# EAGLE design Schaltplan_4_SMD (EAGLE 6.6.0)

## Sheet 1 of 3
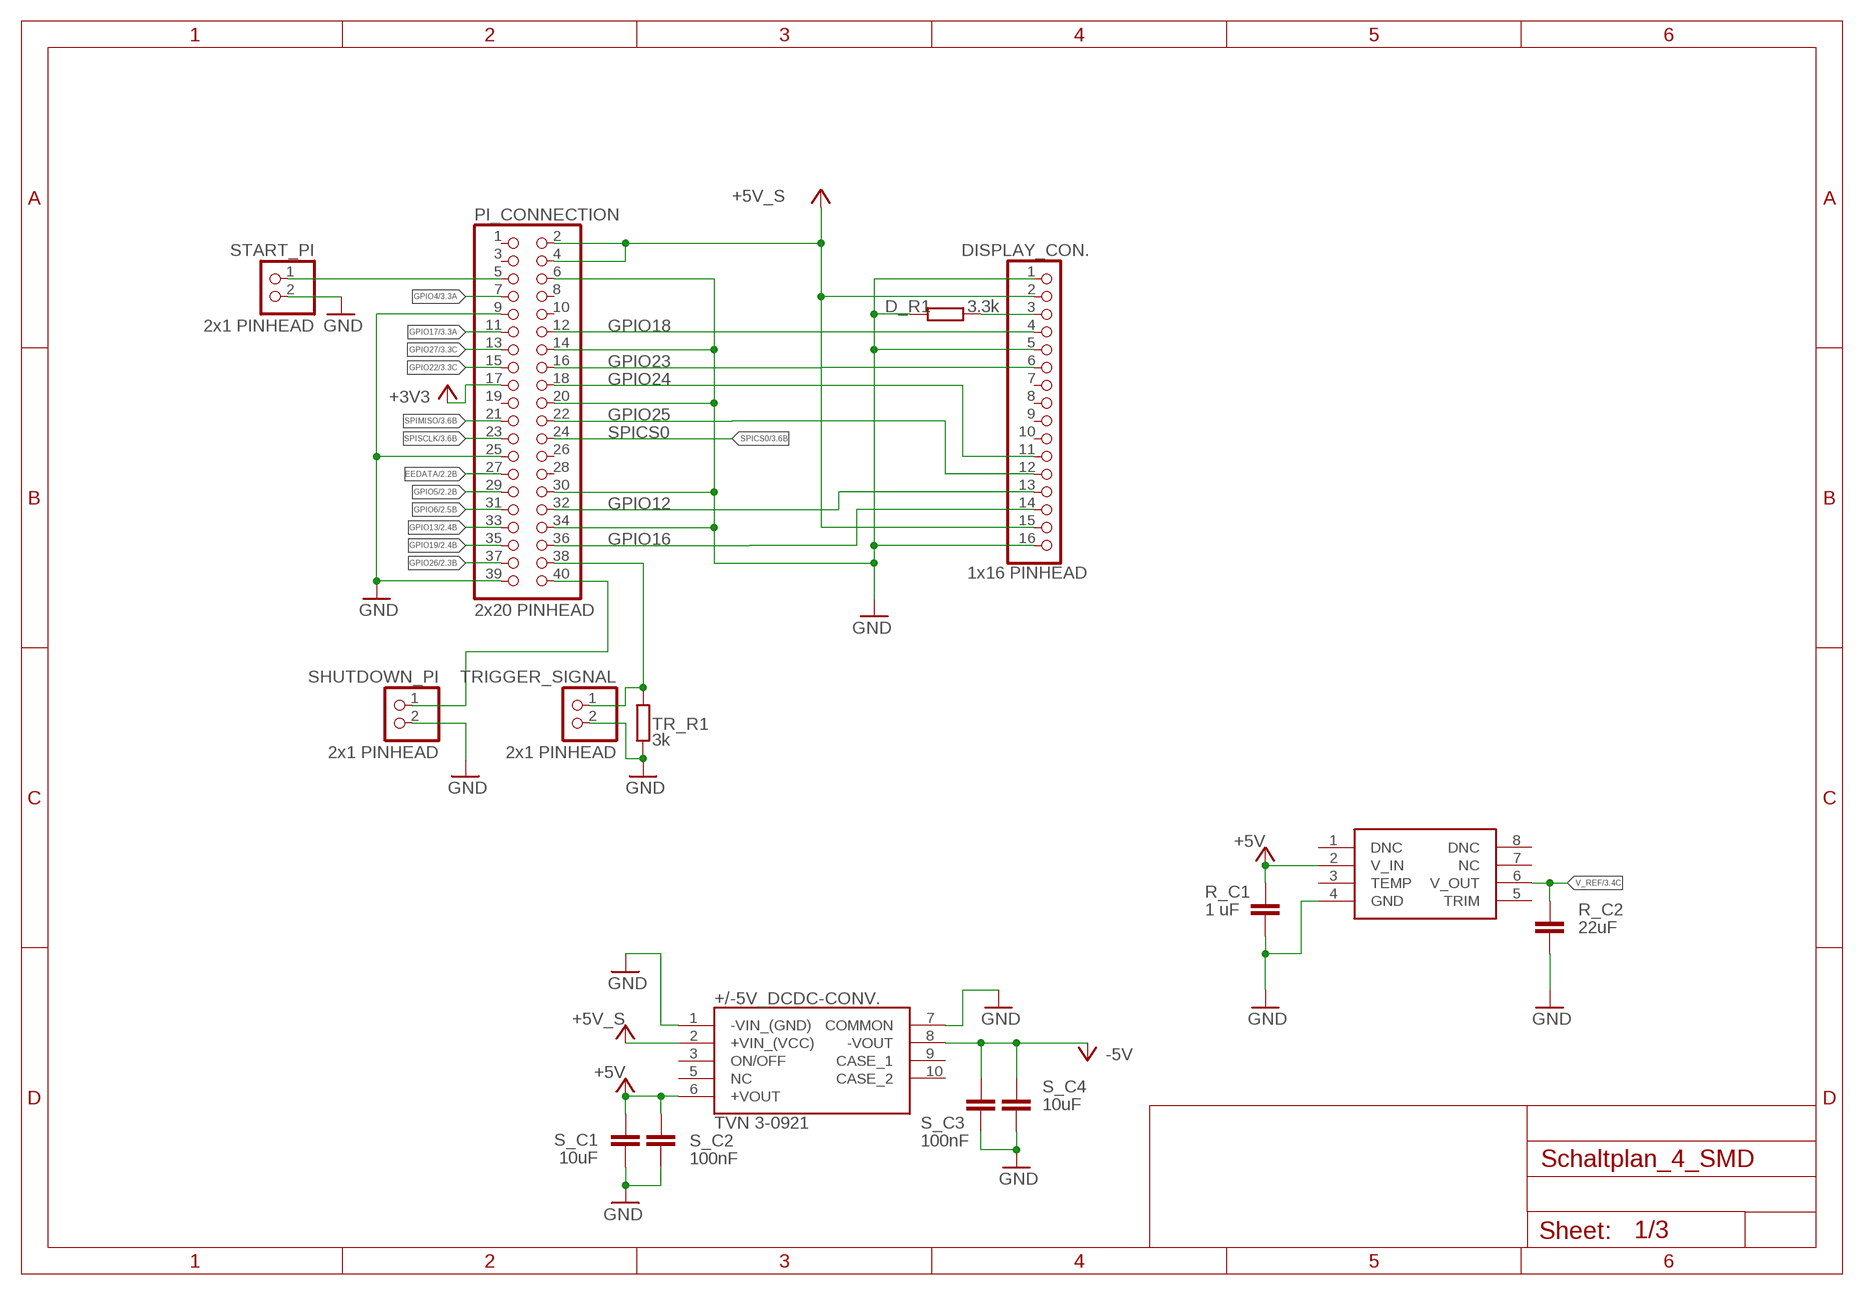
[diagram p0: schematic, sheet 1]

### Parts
+/-5V_DCDC-CONV.  TVN 3-0921  TVN_3-1223  [TVN32419]
D_R1  3.3k  R-EU_0207/10  [0207/10]
DISPLAY_CON.  1x16 PINHEAD  PINHD-1X16  [1X16]
PI_CONNECTION  2x20 PINHEAD  PINHD-2X20  [2X20]
R_C1  1 uF  C-EU025-030X050  [C025-030X050]
R_C2  22uF  C-EU025-030X050  [C025-030X050]
REF_VOLTAGE  REF5020  [SOIC8]
S_C1  10uF  C-EU025-030X050  [C025-030X050]
S_C2  100nF  C-EU025-030X050  [C025-030X050]
S_C3  100nF  C-EU025-030X050  [C025-030X050]
S_C4  10uF  C-EU025-030X050  [C025-030X050]
SHUTDOWN_PI  2x1 PINHEAD  PINHD-1X2  [1X02]
START_PI  2x1 PINHEAD  PINHD-1X2  [1X02]
TR_R1  3k  R-EU_0207/10  [0207/10]
TRIGGER_SIGNAL  2x1 PINHEAD  PINHD-1X2  [1X02]

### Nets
+3V3: PI_CONNECTION.17 ; also sheet 3
+5V: +/-5V_DCDC-CONV..6(+VOUT) R_C1.1 REF_VOLTAGE.2(V_IN) S_C1.1 S_C2.1 ; also sheet 2,3
+5V_SUPPLY: +/-5V_DCDC-CONV..2(+VIN_(VCC)) DISPLAY_CON..2 DISPLAY_CON..15 PI_CONNECTION.2 PI_CONNECTION.4 ; supply symbol labelled +5V_S
-5V: +/-5V_DCDC-CONV..8(-VOUT) S_C3.1 S_C4.2 ; also sheet 2,3
EEDATA: PI_CONNECTION.27 ; also sheet 2
GND: +/-5V_DCDC-CONV..1(-VIN_(GND)) +/-5V_DCDC-CONV..7(COMMON) D_R1.1 DISPLAY_CON..1 DISPLAY_CON..5 DISPLAY_CON..16 PI_CONNECTION.6 PI_CONNECTION.9 PI_CONNECTION.14 PI_CONNECTION.20 PI_CONNECTION.25 PI_CONNECTION.30 PI_CONNECTION.34 PI_CONNECTION.39 R_C1.2 R_C2.2 REF_VOLTAGE.4(GND) S_C1.2 S_C2.2 S_C3.2 S_C4.1 SHUTDOWN_PI.2 START_PI.2 TR_R1.1 TRIGGER_SIGNAL.2 ; also sheet 2,3
GPIO4: PI_CONNECTION.7 ; also sheet 3
GPIO5: PI_CONNECTION.29 ; also sheet 2
GPIO6: PI_CONNECTION.31 ; also sheet 2
GPIO12: DISPLAY_CON..13 PI_CONNECTION.32
GPIO13: PI_CONNECTION.33 ; also sheet 2
GPIO16: DISPLAY_CON..14 PI_CONNECTION.36
GPIO17: PI_CONNECTION.11 ; also sheet 3
GPIO18: DISPLAY_CON..4 PI_CONNECTION.12
GPIO19: PI_CONNECTION.35 ; also sheet 2
GPIO20: PI_CONNECTION.38 TR_R1.2 TRIGGER_SIGNAL.1
GPIO21: PI_CONNECTION.40 SHUTDOWN_PI.1
GPIO22: PI_CONNECTION.15 ; also sheet 3
GPIO23: DISPLAY_CON..6 PI_CONNECTION.16
GPIO24: DISPLAY_CON..11 PI_CONNECTION.18
GPIO25: DISPLAY_CON..12 PI_CONNECTION.22
GPIO26: PI_CONNECTION.37 ; also sheet 2
GPIO27: PI_CONNECTION.13 ; also sheet 3
N$3: D_R1.2 DISPLAY_CON..3
SCL1: PI_CONNECTION.5 START_PI.1
SPICS0: PI_CONNECTION.24 ; also sheet 3
SPIMISO: PI_CONNECTION.21 ; also sheet 3
SPISCLK: PI_CONNECTION.23 ; also sheet 3
V_REF: R_C2.1 REF_VOLTAGE.6(V_OUT) ; also sheet 3
Unconnected: +/-5V_DCDC-CONV..3(ON/OFF) +/-5V_DCDC-CONV..5(NC) +/-5V_DCDC-CONV..9(CASE_1) +/-5V_DCDC-CONV..10(CASE_2) DISPLAY_CON..7 DISPLAY_CON..8 DISPLAY_CON..9 DISPLAY_CON..10 PI_CONNECTION.1 PI_CONNECTION.3 PI_CONNECTION.8 PI_CONNECTION.10 PI_CONNECTION.19 PI_CONNECTION.26 PI_CONNECTION.28 REF_VOLTAGE.1(DNC) REF_VOLTAGE.3(TEMP) REF_VOLTAGE.5(TRIM) REF_VOLTAGE.7(NC) REF_VOLTAGE.8(DNC)

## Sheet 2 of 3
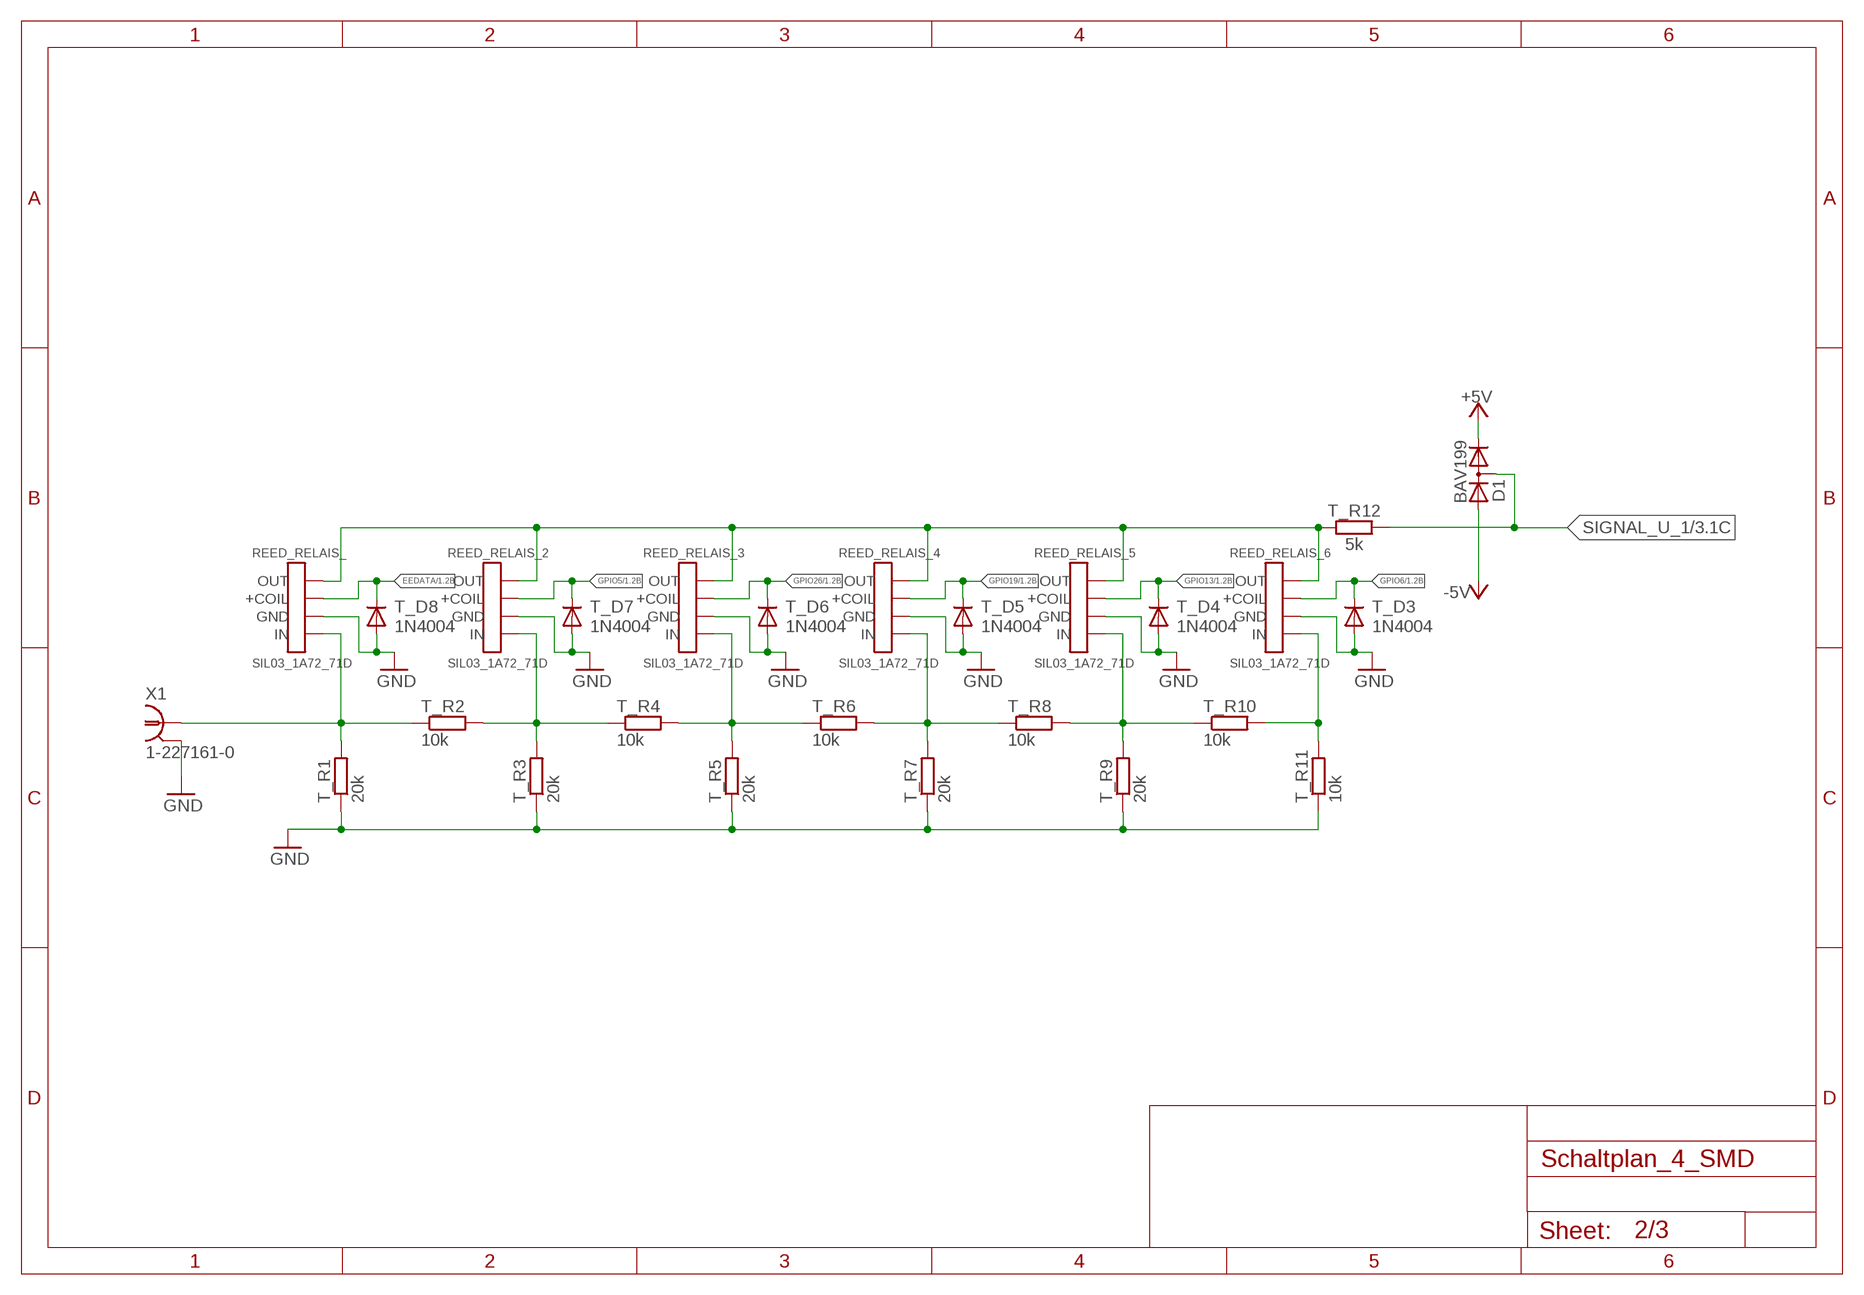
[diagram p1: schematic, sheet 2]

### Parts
D1  BAV199  [SOT23]
REED_RELAIS_  SIL03_1A72_71D  REED_REALIS_SIL03_1A72_71D  [REED_RELAIS_SIL03_1A72_71D]
REED_RELAIS_2  SIL03_1A72_71D  REED_REALIS_SIL03_1A72_71D  [REED_RELAIS_SIL03_1A72_71D]
REED_RELAIS_3  SIL03_1A72_71D  REED_REALIS_SIL03_1A72_71D  [REED_RELAIS_SIL03_1A72_71D]
REED_RELAIS_4  SIL03_1A72_71D  REED_REALIS_SIL03_1A72_71D  [REED_RELAIS_SIL03_1A72_71D]
REED_RELAIS_5  SIL03_1A72_71D  REED_REALIS_SIL03_1A72_71D  [REED_RELAIS_SIL03_1A72_71D]
REED_RELAIS_6  SIL03_1A72_71D  REED_REALIS_SIL03_1A72_71D  [REED_RELAIS_SIL03_1A72_71D]
T_D3  1N4004  BAV17  [DO35-10]
T_D4  1N4004  BAV17  [DO35-10]
T_D5  1N4004  BAV17  [DO35-10]
T_D6  1N4004  BAV17  [DO35-10]
T_D7  1N4004  BAV17  [DO35-10]
T_D8  1N4004  BAV17  [DO35-10]
T_R1  20k  R-EU_0207/10  [0207/10]
T_R2  10k  R-EU_0207/10  [0207/10]
T_R3  20k  R-EU_0207/10  [0207/10]
T_R4  10k  R-EU_0207/10  [0207/10]
T_R5  20k  R-EU_0207/10  [0207/10]
T_R6  10k  R-EU_0207/10  [0207/10]
T_R7  20k  R-EU_0207/10  [0207/10]
T_R8  10k  R-EU_0207/10  [0207/10]
T_R9  20k  R-EU_0207/10  [0207/10]
T_R10  10k  R-EU_0207/10  [0207/10]
T_R11  10k  R-EU_0207/10  [0207/10]
T_R12  5k  R-EU_0207/10  [0207/10]
X1  1-227161-0  [AMP_227161]

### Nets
+5V: D1.2(C) ; also sheet 1,3
-5V: D1.1(A) ; also sheet 1,3
EEDATA: REED_RELAIS_.P$2(+COIL) T_D8.C ; also sheet 1
GND: REED_RELAIS_2.P$3(GND) REED_RELAIS_3.P$3(GND) REED_RELAIS_4.P$3(GND) REED_RELAIS_5.P$3(GND) REED_RELAIS_6.P$3(GND) REED_RELAIS_.P$3(GND) T_D3.A T_D4.A T_D5.A T_D6.A T_D7.A T_D8.A T_R1.1 T_R3.1 T_R5.1 T_R7.1 T_R9.1 T_R11.1 X1.2 ; also sheet 1,3
GPIO5: REED_RELAIS_2.P$2(+COIL) T_D7.C ; also sheet 1
GPIO6: REED_RELAIS_6.P$2(+COIL) T_D3.C ; also sheet 1
GPIO13: REED_RELAIS_5.P$2(+COIL) T_D4.C ; also sheet 1
GPIO19: REED_RELAIS_4.P$2(+COIL) T_D5.C ; also sheet 1
GPIO26: REED_RELAIS_3.P$2(+COIL) T_D6.C ; also sheet 1
N$2: REED_RELAIS_2.P$1(OUT) REED_RELAIS_3.P$1(OUT) REED_RELAIS_4.P$1(OUT) REED_RELAIS_5.P$1(OUT) REED_RELAIS_6.P$1(OUT) REED_RELAIS_.P$1(OUT) T_R12.1
N$42: REED_RELAIS_2.P$4(IN) T_R2.2 T_R3.2 T_R4.1
N$43: REED_RELAIS_3.P$4(IN) T_R4.2 T_R5.2 T_R6.1
N$44: REED_RELAIS_4.P$4(IN) T_R6.2 T_R7.2 T_R8.1
N$45: REED_RELAIS_5.P$4(IN) T_R8.2 T_R9.2 T_R10.1
N$46: REED_RELAIS_6.P$4(IN) T_R10.2 T_R11.2
SIGNAL_U_0: REED_RELAIS_.P$4(IN) T_R1.2 T_R2.1 X1.1
SIGNAL_U_1: D1.3(AC) T_R12.2 ; also sheet 3

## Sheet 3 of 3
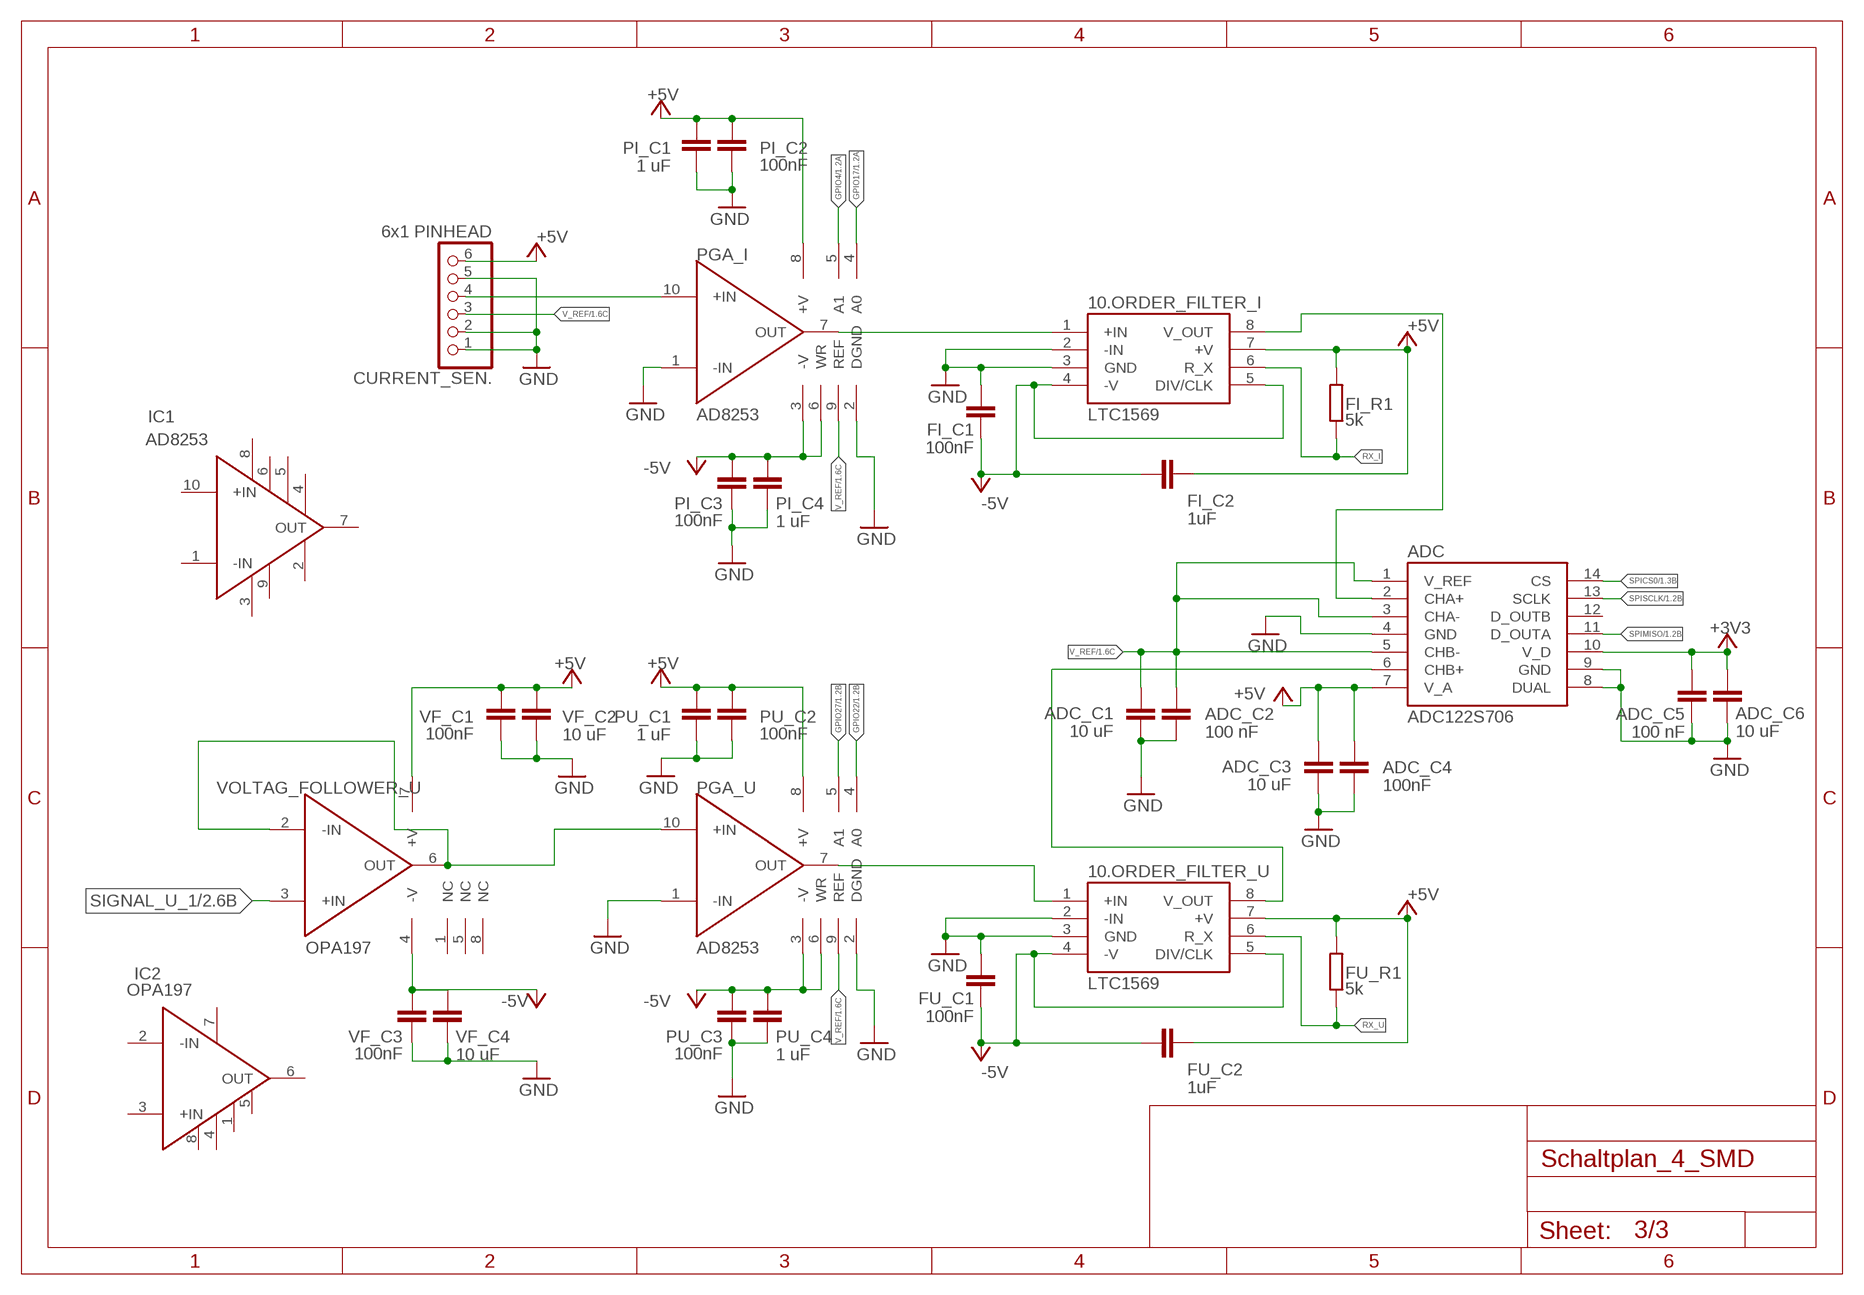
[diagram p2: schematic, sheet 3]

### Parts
10.ORDER_FILTER_I  LTC1569  [SO-08]
10.ORDER_FILTER_U  LTC1569  [SO-08]
ADC  ADC122S706  [TSSOP14]
ADC_C1  10 uF  C-EU025-030X050  [C025-030X050]
ADC_C2  100 nF  C-EU025-030X050  [C025-030X050]
ADC_C3  10 uF  C-EU025-030X050  [C025-030X050]
ADC_C4  100nF  C-EU025-030X050  [C025-030X050]
ADC_C5  100 nF  C-EU025-030X050  [C025-030X050]
ADC_C6  10 uF  C-EU025-030X050  [C025-030X050]
CURRENT_SEN.  6x1 PINHEAD  PINHD-1X6  [1X06]
FI_C1  100nF  C-EU025-030X050  [C025-030X050]
FI_C2  1uF  C-EU025-030X050  [C025-030X050]
FI_R1  5k  R-EU_0207/10  [0207/10]
FU_C1  100nF  C-EU025-030X050  [C025-030X050]
FU_C2  1uF  C-EU025-030X050  [C025-030X050]
FU_R1  5k  R-EU_0207/10  [0207/10]
IC1  AD8253  [MSOP10]
IC2  OPA197  [UMAX8]
PGA_I  AD8253  [MSOP10]
PGA_U  AD8253  [MSOP10]
PI_C1  1 uF  C-EU025-030X050  [C025-030X050]
PI_C2  100nF  C-EU025-030X050  [C025-030X050]
PI_C3  100nF  C-EU025-030X050  [C025-030X050]
PI_C4  1 uF  C-EU025-030X050  [C025-030X050]
PU_C1  1 uF  C-EU025-030X050  [C025-030X050]
PU_C2  100nF  C-EU025-030X050  [C025-030X050]
PU_C3  100nF  C-EU025-030X050  [C025-030X050]
PU_C4  1 uF  C-EU025-030X050  [C025-030X050]
VF_C1  100nF  C-EU025-030X050  [C025-030X050]
VF_C2  10 uF  C-EU025-030X050  [C025-030X050]
VF_C3  100nF  C-EU025-030X050  [C025-030X050]
VF_C4  10 uF  C-EU025-030X050  [C025-030X050]
VOLTAG_FOLLOWER_U  OPA197  [UMAX8]

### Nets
+3V3: ADC.10(V_D) ADC_C5.1 ADC_C6.1 ; also sheet 1
+5V: 10.ORDER_FILTER_I.7(+V) 10.ORDER_FILTER_U.7(+V) ADC.7(V_A) ADC_C3.1 ADC_C4.1 CURRENT_SEN..6 FI_C2.2 FI_R1.2 FU_C2.2 FU_R1.2 PGA_I.8(+V) PGA_U.8(+V) PI_C1.2 PI_C2.1 PU_C1.2 PU_C2.1 VF_C1.1 VF_C2.2 VOLTAG_FOLLOWER_U.7(+V) ; also sheet 1,2
-5V: 10.ORDER_FILTER_I.4(-V) 10.ORDER_FILTER_I.5(DIV/CLK) 10.ORDER_FILTER_U.4(-V) 10.ORDER_FILTER_U.5(DIV/CLK) FI_C1.1 FI_C2.1 FU_C1.1 FU_C2.1 PGA_I.3(-V) PGA_I.6(WR) PGA_U.3(-V) PGA_U.6(WR) PI_C3.1 PI_C4.2 PU_C3.1 PU_C4.2 VF_C3.1 VF_C4.2 VOLTAG_FOLLOWER_U.4(-V) ; also sheet 1,2
GND: 10.ORDER_FILTER_I.2(-IN) 10.ORDER_FILTER_I.3(GND) 10.ORDER_FILTER_U.2(-IN) 10.ORDER_FILTER_U.3(GND) ADC.4(GND) ADC.8(DUAL) ADC.9(GND) ADC_C1.2 ADC_C2.2 ADC_C3.2 ADC_C4.2 ADC_C5.2 ADC_C6.2 CURRENT_SEN..1 CURRENT_SEN..2 CURRENT_SEN..5 FI_C1.2 FU_C1.2 PGA_I.1(-IN) PGA_I.2(DGND) PGA_U.1(-IN) PGA_U.2(DGND) PI_C1.1 PI_C2.2 PI_C3.2 PI_C4.1 PU_C1.1 PU_C2.2 PU_C3.2 PU_C4.1 VF_C1.2 VF_C2.1 VF_C3.2 VF_C4.1 ; also sheet 1,2
GPIO4: PGA_I.5(A1) ; also sheet 1
GPIO17: PGA_I.4(A0) ; also sheet 1
GPIO22: PGA_U.4(A0) ; also sheet 1
GPIO27: PGA_U.5(A1) ; also sheet 1
RX_I: 10.ORDER_FILTER_I.6(R_X) FI_R1.1
RX_U: 10.ORDER_FILTER_U.6(R_X) FU_R1.1
SIGNAL_I_0: CURRENT_SEN..4 PGA_I.10(+IN)
SIGNAL_I_1: 10.ORDER_FILTER_I.1(+IN) PGA_I.7(OUT)
SIGNAL_I_2: 10.ORDER_FILTER_I.8(V_OUT) ADC.2(CHA+)
SIGNAL_U_1: VOLTAG_FOLLOWER_U.3(+IN) ; also sheet 2
SIGNAL_U_2: PGA_U.10(+IN) VOLTAG_FOLLOWER_U.2(-IN) VOLTAG_FOLLOWER_U.6(OUT)
SIGNAL_U_3: 10.ORDER_FILTER_U.1(+IN) PGA_U.7(OUT)
SIGNAL_U_4: 10.ORDER_FILTER_U.8(V_OUT) ADC.6(CHB+)
SPICS0: ADC.14(CS) ; also sheet 1
SPIMISO: ADC.11(D_OUTA) ; also sheet 1
SPISCLK: ADC.13(SCLK) ; also sheet 1
V_REF: ADC.1(V_REF) ADC.3(CHA-) ADC.5(CHB-) ADC_C1.1 ADC_C2.1 CURRENT_SEN..3 PGA_I.9(REF) PGA_U.9(REF) ; also sheet 1
Unconnected: ADC.12(D_OUTB) IC1.1(-IN) IC1.4(A0) IC1.5(A1) IC1.6(WR) IC1.7(OUT) IC1.9(REF) IC1.10(+IN) IC2.1(NC) IC2.2(-IN) IC2.3(+IN) IC2.5(NC) IC2.6(OUT) IC2.8(NC) VOLTAG_FOLLOWER_U.1(NC) VOLTAG_FOLLOWER_U.5(NC) VOLTAG_FOLLOWER_U.8(NC)

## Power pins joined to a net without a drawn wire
+V: IC1.8(+V) IC2.7(+V)
-V: IC1.3(-V) IC2.4(-V)
DGND: IC1.2(DGND)

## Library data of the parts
10.ORDER_FILTER_I 10.ORDER_FILTER_U = ref-packages:LTC1569
+/-5V_DCDC-CONV. = TVN_3-1223:TVN_3-1223: Isolated DC/DC Converters 3W 9-18Vin SIP-8 +/-15Vout +/-100mA Source: Datasheet; ALLIED_NUMBER: 71099550; ALLIED_PRICE-STOCK: https://www.alliedelec.com/traco-power-tvn-3-1223/71099550/; DESCRIPTION: Isolated DC/DC Converters 3W 9-18Vin SIP-8 +/-15Vout +/-100mA; HEIGHT: 11mm; MANUFACTURER_NAME: Traco Power; MANUFACTURER_PART_NUMBER: TVN 3-1223; MOUSER_PART_NUMBER: 495-TVN3-1223; MOUSER_PRICE-STOCK: https://www.mouser.com/Search/Refine.aspx?Keyword=495-TVN3-1223; RS_PART_NUMBER: 1466094; RS_PRICE-STOCK: https://uk.rs-online.com/web/p/products/1466094
ADC = ref-packages:ADC122S706
ADC_C1-ADC_C6 FI_C1 FI_C2 FU_C1 FU_C2 PI_C1-PI_C4 PU_C1-PU_C4 R_C1 R_C2 S_C1-S_C4 VF_C1-VF_C4 = rcl:C-EU: CAPACITOR, European symbol
CURRENT_SEN. = pinhead:PINHD-1X6: PIN HEADER
D1 = diode:BAV199: DIODE low-leakage double diode
D_R1 FI_R1 FU_R1 T_R1-T_R12 TR_R1 = rcl:R-EU_: RESISTOR, European symbol
DISPLAY_CON. = pinhead:PINHD-1X16: PIN HEADER
IC1 = Schaltplan_4_SMD:AD8253
IC2 = Schaltplan_4_SMD:OPA197
PGA_I PGA_U = ref-packages:AD8253
PI_CONNECTION = pinhead:PINHD-2X20: PIN HEADER
REED_RELAIS_ REED_RELAIS_2-REED_RELAIS_6 = OWN_Library:REED_REALIS_SIL03_1A72_71D
REF_VOLTAGE = ref-packages:REF5020
SHUTDOWN_PI START_PI TRIGGER_SIGNAL = pinhead:PINHD-1X2: PIN HEADER
T_D3-T_D8 = diode:BAV17: DIODE
VOLTAG_FOLLOWER_U = ref-packages:OPA197
X1 = con-coax:?227161*: JACK, RIGHT ANGLE, 50 OHM, PCB, BNC; MF: TYCO ELECTRONICS; MPN: 1-227161; OC_FARNELL: unknown; OC_NEWARK: 33B3200

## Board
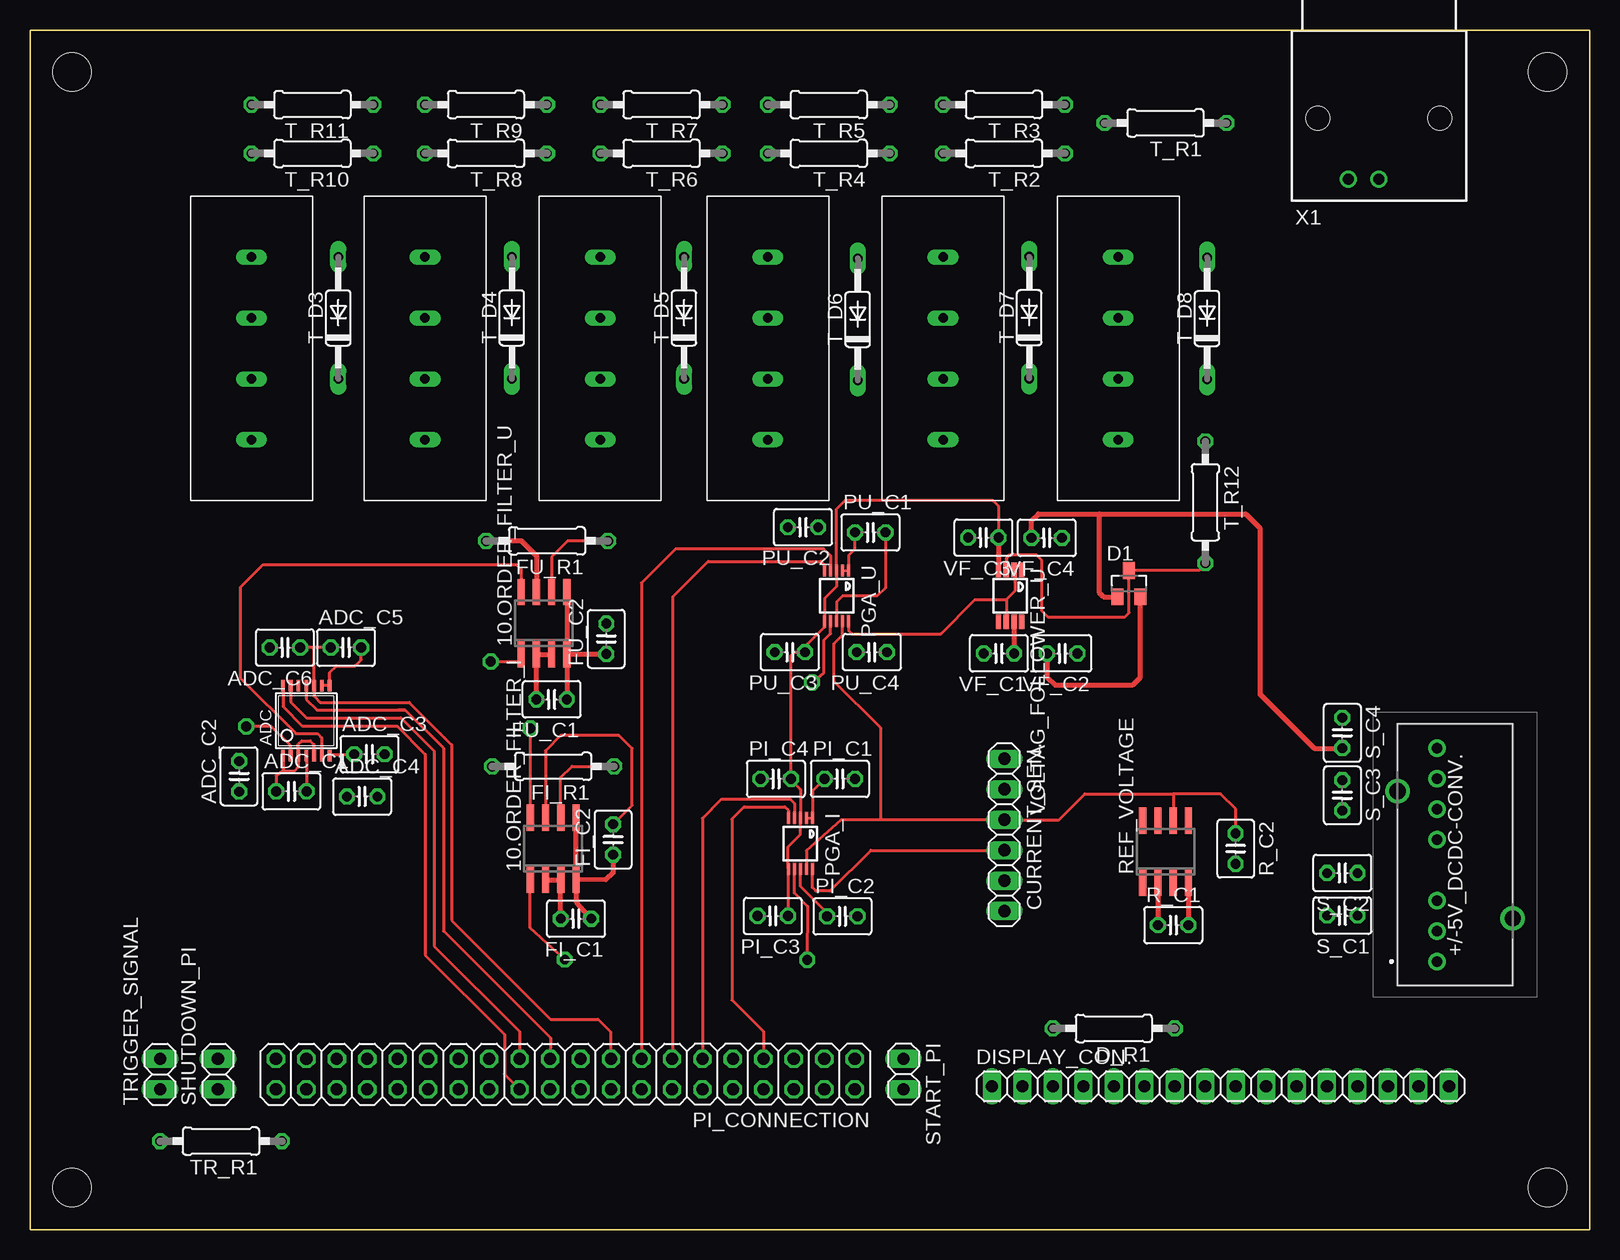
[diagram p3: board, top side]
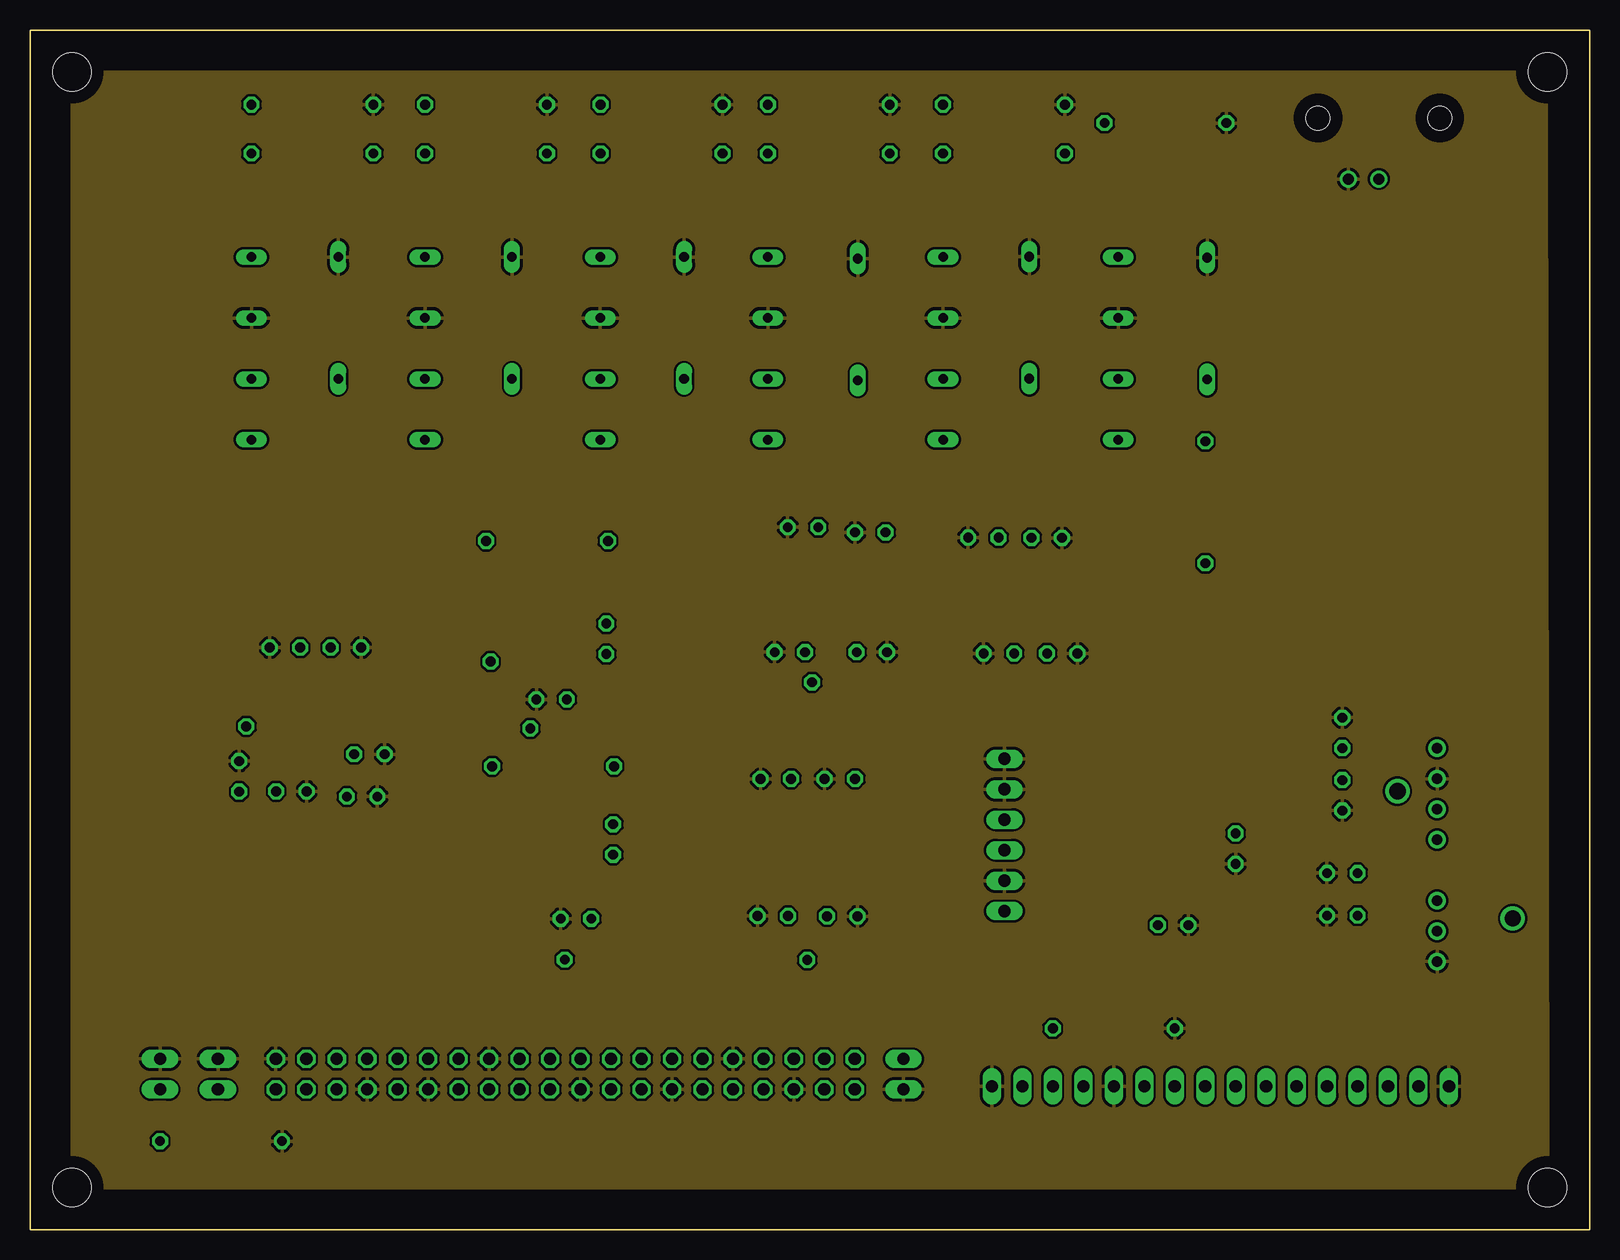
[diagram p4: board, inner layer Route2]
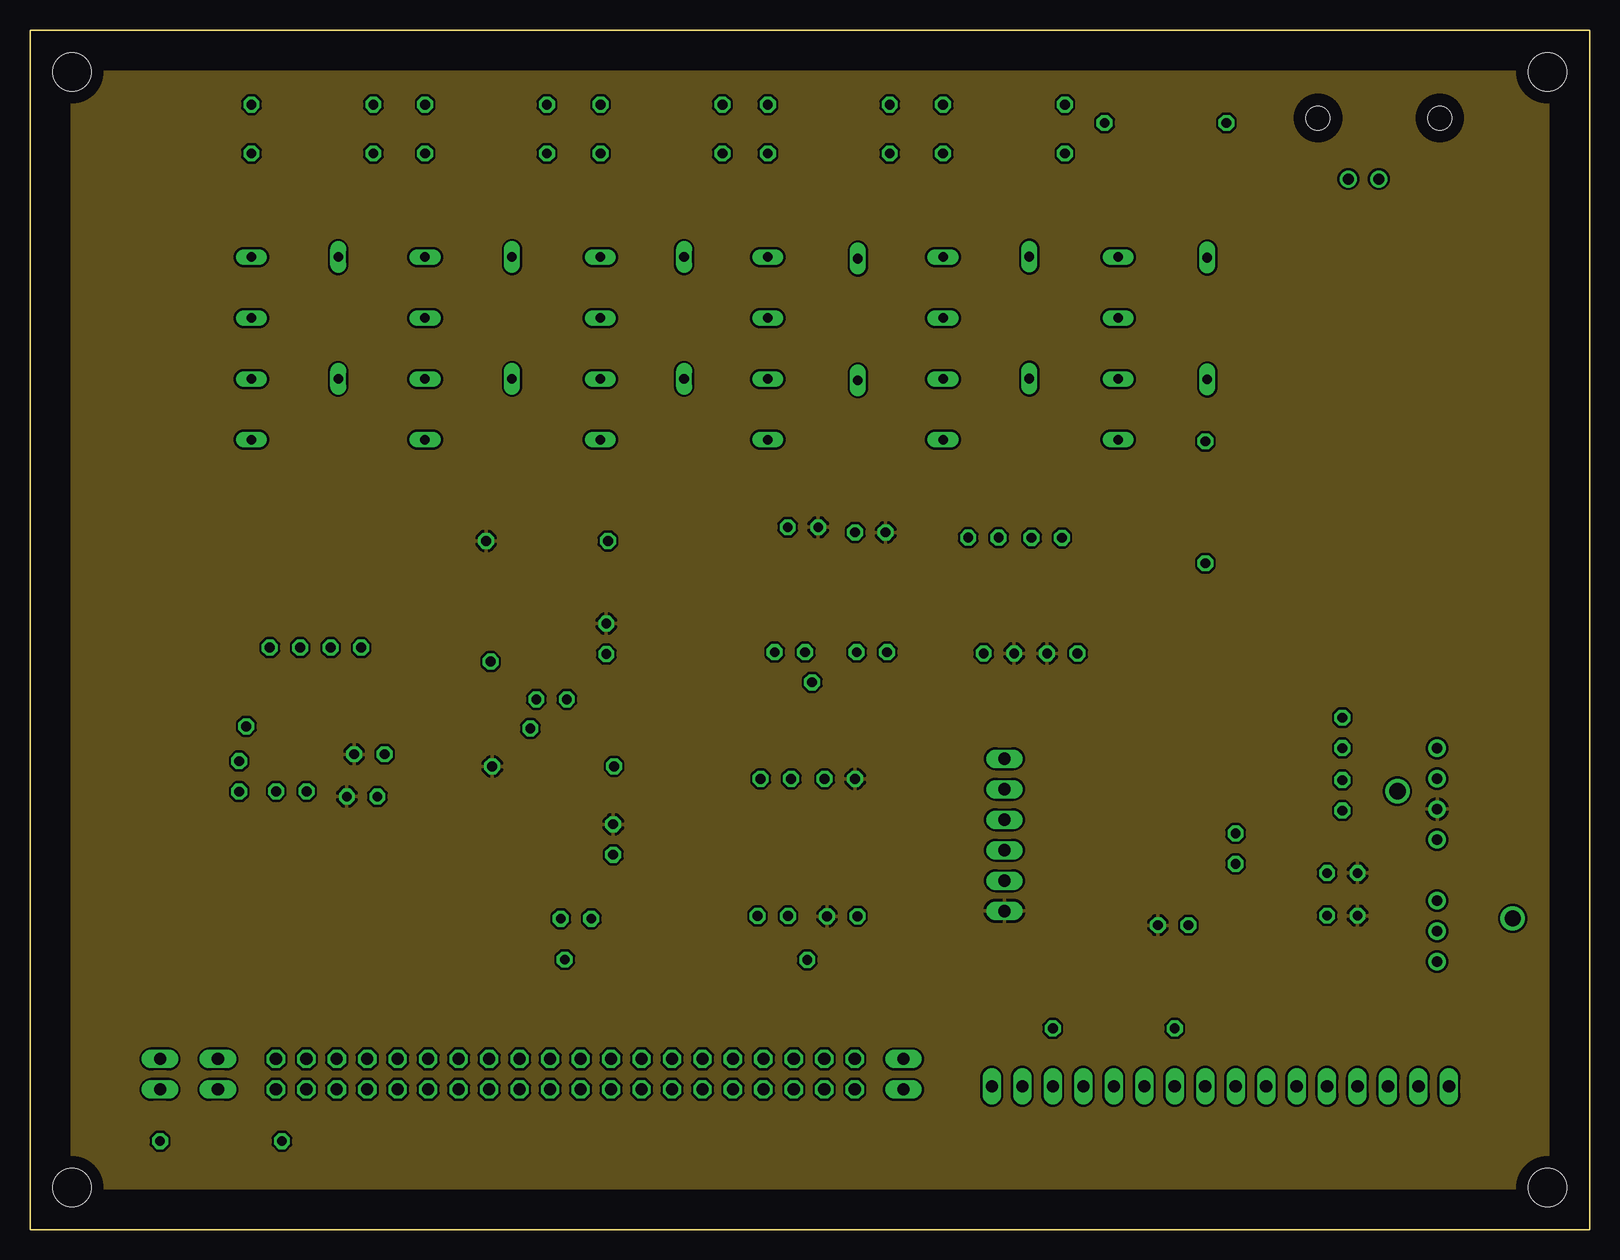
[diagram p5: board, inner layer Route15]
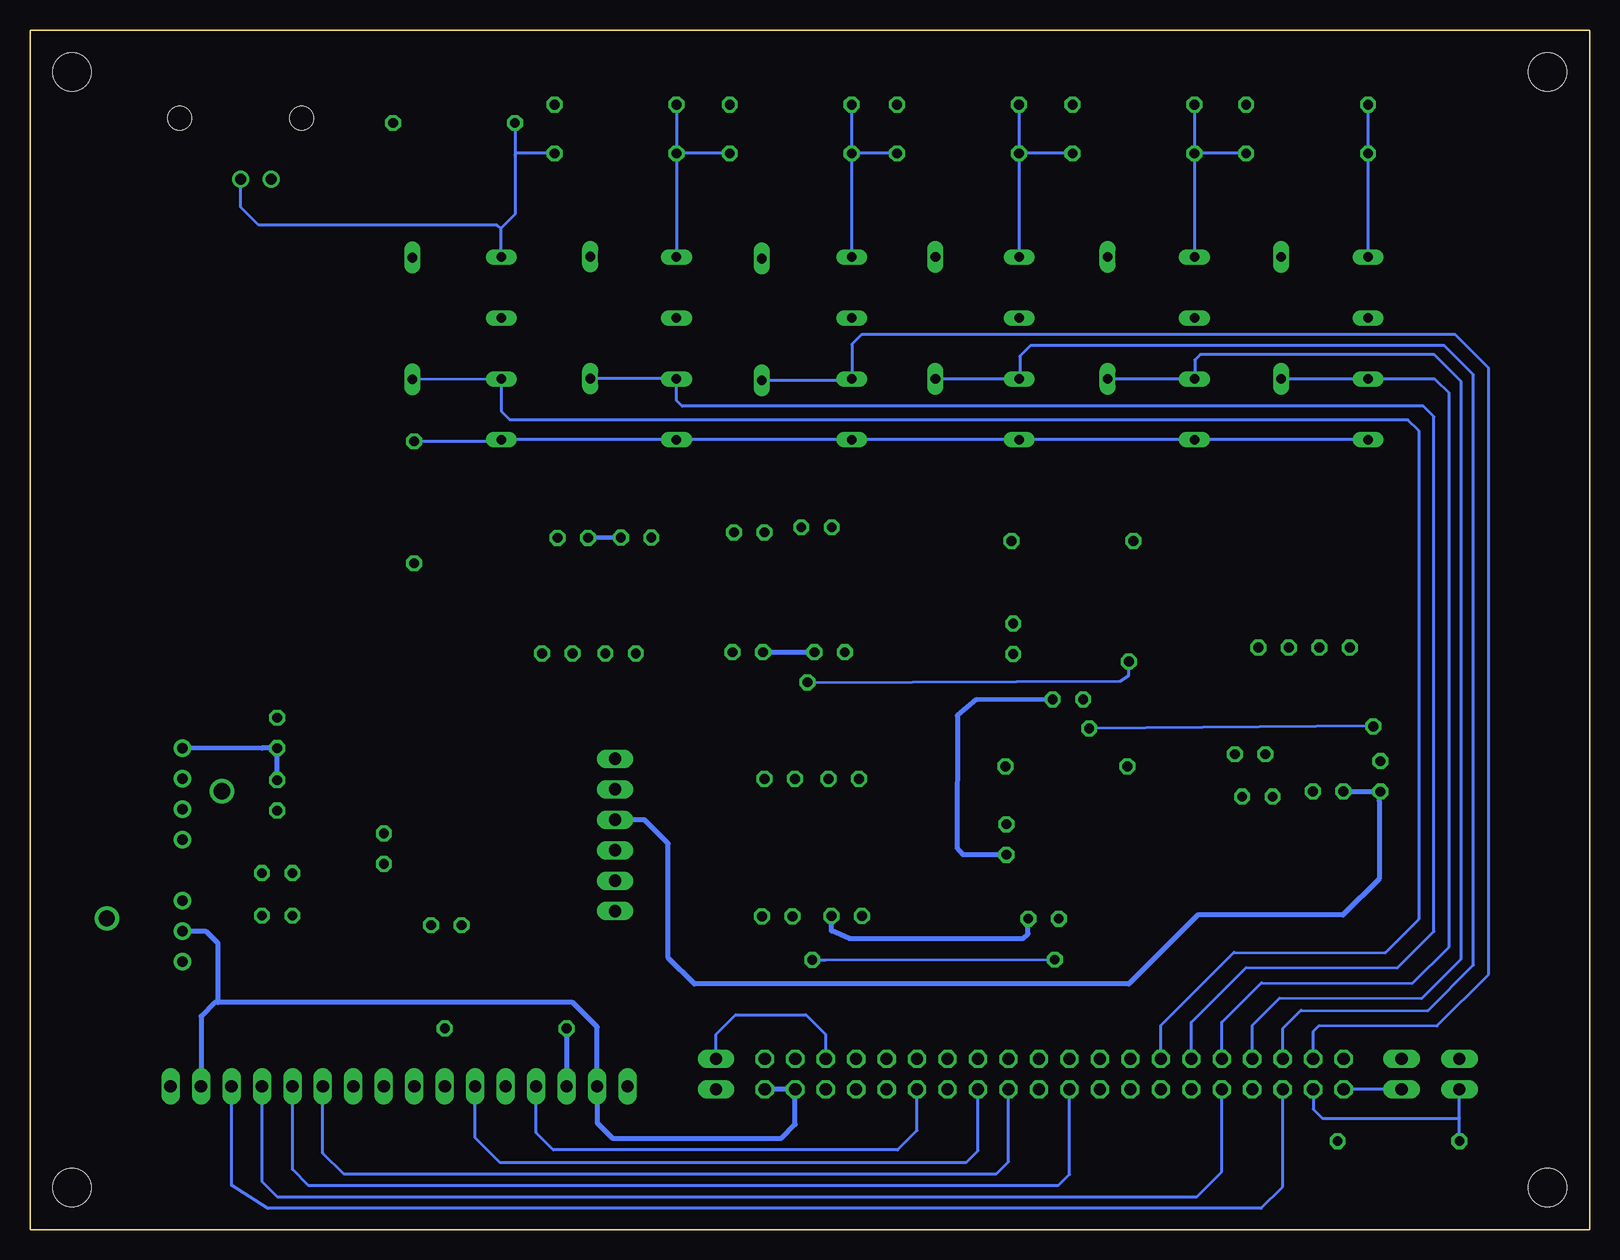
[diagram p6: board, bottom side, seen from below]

Size 130 x 100 mm. Coordinates in mm from the lower left corner, seen from the top.
Outline: 0,0 0,100 130,100 130,0 0,0
Copper layers ((1*2)+(15*16)): Top 0.035mm / dielectric 0.3mm / Route2 0.035mm / dielectric 0.3mm / Route15 0.035mm / dielectric 0.3mm / Bottom 0.035mm
Design rules "default *": minimum track width 10mil, minimum drill 24mil, track to track 8mil, track to pad 2mil, pad to pad 2mil, via to via 8mil, smd to smd 2mil, copper to edge 40mil, drill to drill 8mil, minimum pad ring 10mil, minimum via ring 8mil, stop-mask expansion 4mil, vias tented up to drill 0mil, thermal gap 10mil
Holes 3.2 mm at 3.5,3.5 126.5,96.5 126.5,3.5 3.5,96.5

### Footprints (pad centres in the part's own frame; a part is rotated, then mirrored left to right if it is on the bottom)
SO-08 = smd 0.6 x 2.2: 1 -1.905,-2.6; 2 -0.635,-2.6; 3 0.635,-2.6; 4 1.905,-2.6; 5 1.905,2.6; 6 0.635,2.6; 7 -0.635,2.6; 8 -1.905,2.6
TVN32419 = drill 0.89 pad 1.446: 1 -8.9,1.5; 2 -6.36,1.5; 3 -3.82,1.5; 5 1.26,1.5; 6 3.8,1.5; 7 6.34,1.5; 8 8.88,1.5 | drill 1.35 pad 2.025: 9 -5.3,-4.8; 10 5.3,4.8
TSSOP14 = smd 0.305 x 0.991: 1 -1.95,-2.918; 2 -1.3,-2.918; 3 -0.65,-2.918; 4 0,-2.918; 5 0.65,-2.918; 6 1.3,-2.918; 7 1.95,-2.918; 8 1.95,2.918; 9 1.3,2.918; 10 0.65,2.918; 11 0,2.918; 12 -0.65,2.918; 13 -1.3,2.918; 14 -1.95,2.918
C025-030X050 = drill 0.813 octagon: 1 -1.27,0; 2 1.27,0
1X06 = drill 1.016 long: 1 -6.35,0; 2 -3.81,0; 3 -1.27,0; 4 1.27,0; 5 3.81,0; 6 6.35,0
SOT23 = smd 1 x 1.4: 1 -0.95,-1.1; 2 0.95,-1.1; 3 0,1.1
0207/10 = drill 0.813 octagon: 1 -5.08,0; 2 5.08,0
1X16 = drill 1.016 long: 1 -19.05,0; 2 -16.51,0; 3 -13.97,0; 4 -11.43,0; 5 -8.89,0; 6 -6.35,0; 7 -3.81,0; 8 -1.27,0; 9 1.27,0; 10 3.81,0; 11 6.35,0; 12 8.89,0; 13 11.43,0; 14 13.97,0; 15 16.51,0; 16 19.05,0
MSOP10 = smd 0.25 x 1: 1 -1,-2.113; 2 -0.5,-2.113; 3 0,-2.113; 4 0.5,-2.113; 5 1,-2.113; 6 1,2.113; 7 0.5,2.113; 8 0,2.113; 9 -0.5,2.113; 10 -1,2.113
UMAX8 = smd 0.45 x 1.2: 1 -0.975,-2.175; 2 -0.325,-2.175; 3 0.325,-2.175; 4 0.975,-2.175; 5 0.975,2.175; 6 0.325,2.175; 7 -0.325,2.175; 8 -0.975,2.175
2X20 = drill 1.016 octagon: 1 -24.13,-1.27; 2 -24.13,1.27; 3 -21.59,-1.27; 4 -21.59,1.27; 5 -19.05,-1.27; 6 -19.05,1.27; 7 -16.51,-1.27; 8 -16.51,1.27; 9 -13.97,-1.27; 10 -13.97,1.27; 11 -11.43,-1.27; 12 -11.43,1.27; 13 -8.89,-1.27; 14 -8.89,1.27; 15 -6.35,-1.27; 16 -6.35,1.27; 17 -3.81,-1.27; 18 -3.81,1.27; 19 -1.27,-1.27; 20 -1.27,1.27; 21 1.27,-1.27; 22 1.27,1.27; 23 3.81,-1.27; 24 3.81,1.27; 25 6.35,-1.27; 26 6.35,1.27; 27 8.89,-1.27; 28 8.89,1.27; 29 11.43,-1.27; 30 11.43,1.27; 31 13.97,-1.27; 32 13.97,1.27; 33 16.51,-1.27; 34 16.51,1.27; 35 19.05,-1.27; 36 19.05,1.27; 37 21.59,-1.27; 38 21.59,1.27; 39 24.13,-1.27; 40 24.13,1.27
REED_RELAIS_SIL03_1A72_71D = drill 0.8 long: P$1 0,0; P$2 0,-5.08; P$3 0,-10.16; P$4 0,-15.24
SOIC8 = smd 0.6 x 2.2: 1 -1.905,-2.6; 2 -0.635,-2.6; 3 0.635,-2.6; 4 1.905,-2.6; 5 1.905,2.6; 6 0.635,2.6; 7 -0.635,2.6; 8 -1.905,2.6
1X02 = drill 1.016 long: 1 -1.27,0; 2 1.27,0
DO35-10 = drill 0.813 long: A 5.08,0; C -5.08,0
AMP_227161 = drill 0.9 pad 1.27: 1 0,-5.08; 2 -2.54,-5.08 | hole 2: -5.08,0; 5.08,0

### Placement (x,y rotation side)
10.ORDER_FILTER_I  43.61,31.75 0 top
10.ORDER_FILTER_U  42.85,50.55 0 top
+/-5V_DCDC-CONV.  118.79,31.24 90 top
ADC  23.03,42.42 0 top
ADC_C1  21.79,36.53 0 top
ADC_C2  17.43,37.78 90 top
ADC_C3  28.29,39.62 0 top
ADC_C4  27.68,36.09 0 top
ADC_C5  26.34,48.51 0 top
ADC_C6  21.26,48.51 180 top
CURRENT_SEN.  81.23,32.89 270 top
D1  91.61,53.85 0 top
D_R1  90.34,16.76 180 top
DISPLAY_CON.  99.23,11.94 0 top
FI_C1  45.51,25.91 180 top
FI_C2  48.61,32.51 90 top
FI_R1  43.61,38.61 180 top
FU_C1  43.48,44.2 180 top
FU_C2  48.04,49.24 90 top
FU_R1  43.1,57.4 180 top
IC1  not placed on the board
IC2  not placed on the board
PGA_I  64.21,32.18 180 top
PGA_U  67.23,52.83 180 top
PI_C1  67.51,37.57 0 top
PI_C2  67.71,26.11 0 top
PI_C3  61.92,26.14 180 top
PI_C4  62.18,37.57 0 top
PI_CONNECTION  44.62,12.95 180 top
PU_C1  70.05,58.12 0 top
PU_C2  64.44,58.55 180 top
PU_C3  63.34,48.13 180 top
PU_C4  70.18,48.13 180 top
R_C1  95.3,25.37 0 top
R_C2  100.5,31.75 270 top
REED_RELAIS_  90.72,65.83 180 top
REED_RELAIS_2  76.11,65.83 180 top
REED_RELAIS_3  61.51,65.83 180 top
REED_RELAIS_4  47.54,65.83 180 top
REED_RELAIS_5  32.93,65.83 180 top
REED_RELAIS_6  18.46,65.83 180 top
REF_VOLTAGE  94.66,31.5 0 top
S_C1  109.39,26.16 180 top
S_C2  109.39,29.72 180 top
S_C3  109.39,36.2 270 top
S_C4  109.39,41.4 270 top
SHUTDOWN_PI  15.67,12.95 90 top
START_PI  72.82,12.95 270 top
T_D3  25.7,75.99 90 top
T_D4  40.17,75.99 90 top
T_D5  54.52,75.99 90 top
T_D6  69,75.87 90 top
T_D7  83.3,76.02 90 top
T_D8  98.12,75.95 90 top
T_R1  94.65,92.25 180 top
T_R2  81.19,89.71 180 top
T_R3  81.19,93.77 180 top
T_R4  66.59,89.71 180 top
T_R5  66.59,93.77 180 top
T_R6  52.64,89.71 180 top
T_R7  52.64,93.77 180 top
T_R8  38.01,89.71 180 top
T_R9  38.01,93.77 180 top
T_R10  23.54,89.71 180 top
T_R11  23.54,93.77 180 top
T_R12  97.98,60.63 270 top
TR_R1  15.92,7.37 180 top
TRIGGER_SIGNAL  10.84,12.95 90 top
VF_C1  80.77,48.03 180 top
VF_C2  86.05,48.03 180 top
VF_C3  79.47,57.68 180 top
VF_C4  84.76,57.66 180 top
VOLTAG_FOLLOWER_U  81.71,52.83 180 top
X1  112.44,92.65 0 top

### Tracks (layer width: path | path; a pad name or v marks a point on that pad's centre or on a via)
+3V3
  Top 0.254: ADC_C5.1 23.54,48.51 | 23.54,48.51 ADC_C6.1 | 23.54,48.51 23.68,48.37 ADC.10 23.68,44.46 24.2,43.94 31.62,43.94 35.15,40.41 35.15,28.93 35.15,25.78 43.39,17.54 47.34,17.54 48.4,16.48 48.4,14.26 PI_CONNECTION.17
+5V
  Top 0.254: ADC.7 25.01,39.6 25.02,39.62 ADC_C3.1 | PU_C1.2 71.32,53.49 70.61,52.83 67.74,52.83 67.23,52.33 PGA_U.8 | PI_C2.1 66.44,26.39 64.21,28.63 PGA_I.8 | FI_C2.2 50.19,35.36 50.19,40.11 49.1,41.17 44.25,41.17 42.97,39.9 10.ORDER_FILTER_I.7
  Top 0.406: VOLTAG_FOLLOWER_U.7 VF_C1.1 | VF_C2.2 84.78,46.08 85.47,45.39 91.93,45.4 92.55,46.01 92.55,52.74 D1.2 | REF_VOLTAGE.2 R_C1.1 | FU_R1.2 38.05,57.43 40.94,57.43 42.21,56.16 10.ORDER_FILTER_U.7
  pour Route15: 3.5,3.5 3.5,96.5 126.5,96.5 126.5,3.5
+5V_SUPPLY
  Bottom 0.406: 116,12.19 DISPLAY_CON..15 115.74,17.78 114.6,18.92 114.35,18.92 | PI_CONNECTION.2 PI_CONNECTION.4 66.21,8.76 67.36,7.62 81.45,7.62 82.72,8.89 DISPLAY_CON..2 82.72,16.89 84.76,18.92 114.35,18.92 | +/-5V_DCDC-CONV..2 117.28,24.89 115.36,24.89 114.35,23.88 114.35,18.92
+V  (1 unrouted)
-5V
  Top 0.254: VF_C3.1 80.74,60.3 80.23,60.81 67.97,60.81 67.23,60.07 PGA_U.3 67.23,53.62 66.23,52.62 PGA_U.6 66.24,50.71 66.24,50.22 64.61,48.59 PU_C3.1 63.73,48.13 63.42,47.83 63.42,37.59 PI_C4.2 63.45,37.47 64.24,36.68 64.21,36.65 PGA_I.3 64.21,32.92 63.2,31.9 63.2,30.09 PGA_I.6 63.21,26.16 PI_C3.1
  Top 0.406: 10.ORDER_FILTER_U.4 FU_C1.1 | FI_C1.1 45.56,27.28 10.ORDER_FILTER_I.4 | D1.1 89.48,52.75 89.15,53.07 89.15,59.66 | VF_C4.2 83.49,59.11 84.05,59.66 89.15,59.66 | VF_C3.1 80.73,56.6 VOLTAG_FOLLOWER_U.4 | S_C4.2 109.37,40.11 107.06,40.11 102.54,44.63 102.54,58.47 101.35,59.66 89.15,59.66 | FI_C2.1 48.61,29.74 48.02,29.18 10.ORDER_FILTER_I.4 | 10.ORDER_FILTER_I.4 10.ORDER_FILTER_I.5 | 10.ORDER_FILTER_U.5 10.ORDER_FILTER_U.4 | FU_C2.1 48.01,47.95 10.ORDER_FILTER_U.4
  Bottom 0.406: +/-5V_DCDC-CONV..8 110.68,40.13 S_C4.2 S_C3.1 | VF_C3.1 VF_C4.2 | FI_C1.1 46.81,24.66 47.24,24.26 61.72,24.26 63.17,24.89 63.19,24.92 PI_C3.1 | FU_C1.1 44.8,44.15 51.1,44.17 52.7,42.85 52.73,31.85 52.19,31.24 FI_C2.1 | PU_C4.2 PU_C3.1
-V  (1 unrouted)
EEDATA
  Bottom 0.254: PI_CONNECTION.27 35.73,17.02 29.64,23.11 17.04,23.06 14.25,25.86 14.25,66.6 15.13,67.48 89.98,67.48 90.7,68.2 90.7,70.9 REED_RELAIS_.P$2 90.74,70.89 T_D8.C
GND
  Top 0.254: ADC.9 ADC.8 24.99,46.43 25.55,46.99 27.1,46.99 27.61,47.5 ADC_C5.2 | PU_C1.1 68.73,56.69 68.23,56.2 PGA_U.1 | PI_C1.1 65.21,36.53 PGA_I.1 PGA_I.2 | ADC.4 23.06,39.48 ADC_C1.2 | 68.25,54.96 PGA_U.1 | PGA_U.2 PGA_U.1
  Top 0.406: FU_C1.2 10.ORDER_FILTER_U.2 10.ORDER_FILTER_U.3 | FI_C1.2 10.ORDER_FILTER_I.3 10.ORDER_FILTER_I.2 | REF_VOLTAGE.4 R_C1.2
  pour Route2: 3.5,3.5 3.5,96.5 126.4,96.5 126.5,3.5
GPIO4
  Top 0.254: PI_CONNECTION.7 61.13,16.51 58.52,19.13 58.52,34.23 59.53,35.24 62.94,35.24 63.22,34.96 63.21,34.96 PGA_I.5
GPIO5
  Bottom 0.254: PI_CONNECTION.29 33.19,17.27 28.62,21.84 16.02,21.79 12.98,24.84 12.98,67.76 13.84,68.63 75.63,68.63 76.1,69.1 REED_RELAIS_2.P$2 76.14,70.94 T_D7.C
GPIO6
  Bottom 0.254: PI_CONNECTION.31 30.65,17.27 27.35,20.57 14.75,20.52 11.71,23.57 11.71,69.72 12.9,70.91 REED_RELAIS_6.P$2 T_D3.C
GPIO12
  Bottom 0.254: DISPLAY_CON..13 110.66,3.99 109.37,2.7 32.79,2.7 30.65,4.83 PI_CONNECTION.32
GPIO13
  Bottom 0.254: PI_CONNECTION.33 28.11,17.02 25.83,19.3 13.99,19.25 10.69,22.55 10.69,70.69 12.95,72.95 32.45,72.95 32.9,72.5 32.9,70.95 REED_RELAIS_5.P$2 T_D4.C
GPIO16
  Bottom 0.254: 25.45,11.56 PI_CONNECTION.36 25.57,3.57 27.38,1.76 110.18,1.76 113.2,3.68 DISPLAY_CON..14
GPIO17
  Top 0.254: PI_CONNECTION.11 56.05,34.29 57.65,35.89 63.34,35.89 63.71,35.52 PGA_I.4
GPIO18
  Bottom 0.254: DISPLAY_CON..4 87.8,8.07 86.38,6.64 57.68,6.64 56.05,8.27 PI_CONNECTION.12
GPIO19
  Bottom 0.254: PI_CONNECTION.35 25.57,16.76 24.05,18.29 13.48,18.24 9.67,22.05 9.67,71.27 12.11,73.71 46.59,73.71 47.5,72.8 47.5,70.95 REED_RELAIS_4.P$2 T_D5.C
GPIO20
  Bottom 0.254: TR_R1.2 10.84,9.27 | 10.84,9.27 TRIGGER_SIGNAL.1 | 10.84,9.27 22.27,9.27 23.03,10.03 PI_CONNECTION.38
GPIO21
  Bottom 0.254: SHUTDOWN_PI.1 PI_CONNECTION.40
GPIO22
  Top 0.254: PI_CONNECTION.15 50.97,53.9 53.82,56.74 66.16,56.74 66.73,56.17 PGA_U.4
GPIO23
  Bottom 0.254: DISPLAY_CON..6 92.88,7.64 90.83,5.58 51.96,5.58 50.97,6.57 PI_CONNECTION.16
GPIO24
  Bottom 0.254: DISPLAY_CON..11 105.58,6.37 103.83,4.62 49.48,4.62 48.43,5.66 PI_CONNECTION.18
GPIO25
  Bottom 0.254: DISPLAY_CON..12 108.12,5 106.78,3.66 44.3,3.66 43.35,4.6 PI_CONNECTION.22
GPIO26
  Bottom 0.254: PI_CONNECTION.37 23.03,16.51 22.53,17.02 12.72,16.97 8.4,21.29 8.4,71.83 11.17,74.6 60.7,74.6 61.5,73.8 61.5,70.92 REED_RELAIS_3.P$2 | REED_RELAIS_3.P$2 61.63,70.79 T_D6.C | REED_RELAIS_3.P$2
GPIO27
  Top 0.254: PI_CONNECTION.13 53.56,14.28 53.56,52.73 56.54,55.7 65.93,55.7 66.23,55.4 PGA_U.5
N$2
  Bottom 0.254: REED_RELAIS_6.P$1 REED_RELAIS_5.P$1 REED_RELAIS_4.P$1 REED_RELAIS_3.P$1 REED_RELAIS_2.P$1 REED_RELAIS_.P$1 90.84,65.71 94.7,65.7 96.19,65.71 T_R12.1
N$3
  Bottom 0.406: D_R1.2 DISPLAY_CON..3
N$42
  Bottom 0.254: T_R4.1 T_R2.2 | T_R3.2 T_R2.2 | T_R2.2 REED_RELAIS_2.P$4
N$43
  Bottom 0.254: T_R5.2 T_R4.2 | T_R4.2 REED_RELAIS_3.P$4 | T_R6.1 T_R4.2
N$44
  Bottom 0.254: T_R7.2 T_R6.2 | T_R6.2 47.56,81.1 REED_RELAIS_4.P$4 | T_R8.1 T_R6.2
N$45
  Bottom 0.254: T_R9.2 T_R8.2 | T_R8.2 REED_RELAIS_5.P$4 | T_R10.1 T_R8.2
N$46
  Bottom 0.254: T_R11.2 T_R10.2 REED_RELAIS_6.P$4
RX_I
  Top 0.254: 10.ORDER_FILTER_I.6 44.24,37.67 45.18,38.61 FI_R1.1
RX_U
  Top 0.254: FU_R1.1 48.16,57.38 44.8,57.38 43.48,56.06 10.ORDER_FILTER_U.6
SCL1
  Bottom 0.254: START_PI.1 72.82,16.26 71.17,17.91 65.33,17.91 63.67,16.26 PI_CONNECTION.5
SIGNAL_I_0
  Top 0.254: CURRENT_SEN..4 70.1,31.62 66.7,28.22 65.51,28.22 65.21,28.52 PGA_I.10
SIGNAL_I_1  (via drill 0.81 pad 1.32)
  Top 0.254: v64.79,22.48 64.82,26.95 63.71,28.05 PGA_I.7 | v44.57,22.5 41.7,25.15 10.ORDER_FILTER_I.1
  Bottom 0.254: v64.79,22.48 63.67,22.48 v44.57,22.5
SIGNAL_I_2  (via drill 0.81 pad 1.32)
  Top 0.254: ADC.2 21.71,39.53 21.71,40.34 20.1,41.95 v18.03,41.95 | v41.7,41.77 10.ORDER_FILTER_I.8
  Bottom 0.254: v18.03,41.95 18.06,41.97 v41.7,41.77
SIGNAL_U_0
  Bottom 0.254: T_R1.2 89.57,89.58 | 89.57,89.58 89.57,84.63 90.72,83.49 | T_R2.1 89.45,89.71 89.57,89.58 | REED_RELAIS_.P$4 90.72,83.49 | 90.72,83.49 91.1,83.74 110.93,83.74 112.44,85.23 X1.1
SIGNAL_U_1
  Top 0.254: T_R12.2 97.98,55.48 97.5,55 91.67,55 D1.3 91.61,51.41 91.26,51.05 84.86,51.05 84.32,51.59 84.32,55.8 83.87,56.26 81.71,56.26 81.38,55.94 VOLTAG_FOLLOWER_U.3
SIGNAL_U_2
  Top 0.254: VOLTAG_FOLLOWER_U.2 82.09,54.95 82.09,53.21 81.38,52.51 | 81.38,52.51 VOLTAG_FOLLOWER_U.6 | 81.38,52.51 81.38,52.5 78.76,52.5 75.92,49.66 68.53,49.66 68.25,49.94 68.25,50.7 PGA_U.10
SIGNAL_U_3  (via drill 0.81 pad 1.32)
  Top 0.254: v65.2,45.62 66.16,46.41 66.16,49.1 66.73,49.67 PGA_U.7 | v38.4,47.35 39.08,47.34 40.83,47.34 40.95,47.45 10.ORDER_FILTER_U.1
  Bottom 0.254: v65.2,45.62 65.1,45.62 39.09,45.72 38.4,46.17 v38.4,47.35
SIGNAL_U_4
  Top 0.254: ADC.6 24.33,41 23.97,41.35 22.17,41.35 17.53,45.99 17.53,53.53 19.41,55.41 40.58,55.41 40.94,55.06 10.ORDER_FILTER_U.8
SPICS0
  Top 0.254: ADC.14 21.08,43.61 22.7,41.96 30.6,41.96 32.94,39.62 32.94,22.86 39.54,16.26 39.54,12.95 PI_CONNECTION.24
SPIMISO
  Top 0.254: ADC.11 23.03,44.2 23.92,43.31 30.71,43.33 | 30.71,43.33 31.24,43.33 | PI_CONNECTION.21 43.38,15.98 34.46,24.89 34.46,40.13 31.27,43.33 30.71,43.33
SPISCLK
  Top 0.254: ADC.13 21.73,43.97 23.06,42.65 30.93,42.65 33.7,39.88 33.7,23.62 40.81,16.51 PI_CONNECTION.23
V_REF
  Top 0.254: ADC.1 21.08,38.31 21.08,38.2 | 21.08,38.2 20.52,37.84 20.51,36.49 ADC_C1.1 | R_C2.1 100.5,35.05 99.23,36.32 95.3,36.32 | 95.3,36.32 REF_VOLTAGE.6 | 95.3,36.32 87.93,36.32 85.77,34.16 CURRENT_SEN..3 70.89,34.16 | 21.08,38.2 22.02,38.2 22.37,38.56 ADC.3 22.37,39.51 22.37,40.46 22.65,40.74 23.36,40.74 23.66,40.45 23.66,40.4 ADC.5 | 70.89,34.16 67.61,34.16 64.72,31.59 64.71,31.59 PGA_I.9 | 70.89,34.16 70.89,41.83 67.03,45.7 67.03,48.84 67.73,49.55 PGA_U.9
  Bottom 0.254: ADC_C2.1 17.52,35.74
  Bottom 0.406: ADC_C1.1 ADC_C2.1 | 17.52,35.74 17.52,29.23 20.55,26.21 32.66,26.21 38.4,20.47 74.62,20.47 76.81,22.66 76.81,32.18 78.79,34.16 CURRENT_SEN..3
